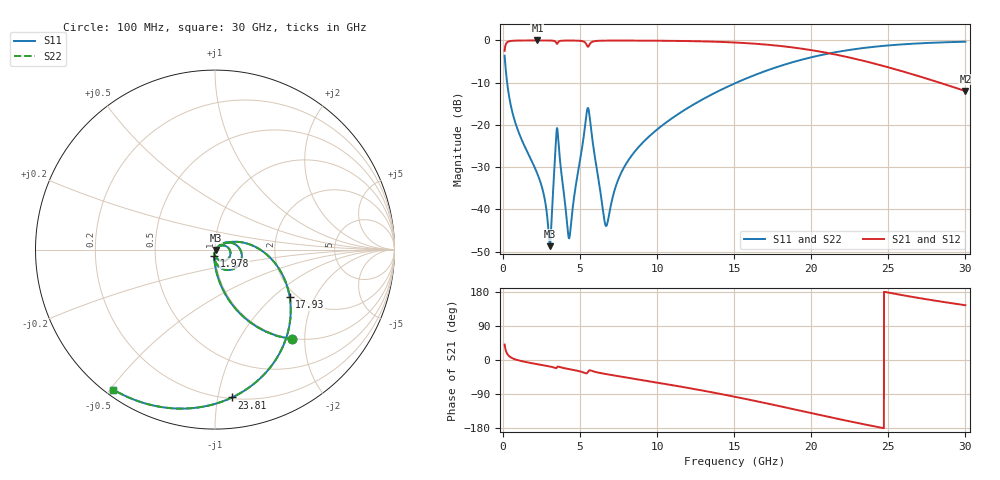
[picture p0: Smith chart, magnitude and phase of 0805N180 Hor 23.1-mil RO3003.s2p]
# GHz S MA R 50
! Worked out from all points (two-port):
!   3201 points, 100 MHz to 30 GHz, reference 50 ohm
!   highest |S21| = -0.02 dB at 2.23 GHz (marker M1); lowest = -12.0 dB at 30 GHz (marker M2)
!   |S21| within 3 dB of the highest: start of sweep to 21.11 GHz
!   lowest |S11| = -48.7 dB at 3.034 GHz (marker M3), VSWR 1.01, Z = 50.3 - j0.179 ohm
!   |S11| at or under -10 dB: 261.9 MHz to 15.15 GHz (14.89 GHz wide, 193 % of centre)
!   |S22| runs from -48.7 to -0.3 dB; largest |S21 - S12| = 0
!   S11 on the Smith chart (normalised r, x): 100 MHz: 0.98, -1.74; 1.978 GHz: 0.99, -0.07; 17.93 GHz: 1.84, -1.29; 23.81 GHz: 0.21, -1.10; 30 GHz: 0.02, -0.51
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0.1  0.6588 -49.3  0.752 40.6  0.752 40.6  0.6588 -49.3
0.3335938  0.2527 -77.1  0.967 12.7  0.967 12.7  0.2527 -77.1
0.7073438  0.1198 -86.7  0.9919 2.9  0.9919 2.9  0.1198 -86.7
1.978094  0.03354 -96.7  0.9978 -9.3  0.9978 -9.3  0.03354 -96.7
2.230375  0.02625 -97.4  0.9979 -11.1  0.9979 -11.1  0.02625 -97.4
3.033937  0.003665 -29.0  0.9963 -17.1  0.9963 -17.1  0.003665 -29.0
3.398344  0.05028 27.5  0.9661 -21.3  0.9661 -21.3  0.05028 27.5
3.501125  0.09161 -23.8  0.9085 -19.3  0.9085 -19.3  0.09161 -23.8
4.276656  0.004545 -26.6  0.9953 -24.0  0.9953 -24.0  0.004545 -26.6
5.089563  0.04838 40.8  0.9838 -31.1  0.9838 -31.1  0.04838 40.8
5.40725  0.1316 6.1  0.8972 -35.2  0.8972 -35.2  0.1316 6.1
5.55675  0.1494 -46.1  0.8564 -28.5  0.8564 -28.5  0.1494 -46.1
6.519156  0.008698 -71.0  0.9926 -36.0  0.9926 -36.0  0.008698 -71.0
6.706031  0.00637 -25.0  0.9935 -37.3  0.9935 -37.3  0.00637 -25.0
7.845969  0.03134 36.4  0.9946 -45.1  0.9946 -45.1  0.03134 36.4
10.06978  0.09037 27.0  0.9909 -60.0  0.9909 -60.0  0.09037 27.0
15.05  0.3105 -8.3  0.9435 -97.1  0.9435 -97.1  0.3105 -8.3
17.92788  0.4939 -32.5  0.861 -121.6  0.861 -121.6  0.4939 -32.5
20.03956  0.6331 -51.2  0.7646 -140.5  0.7646 -140.5  0.6331 -51.2
23.80509  0.8293 -83.4  0.5481 -172.8  0.5481 -172.8  0.8293 -83.4
25.01978  0.8719 -92.9  0.4786 177.7  0.4786 177.7  0.8719 -92.9
30  0.9644 -126.0  0.2512 144.5  0.2512 144.5  0.9644 -126.0
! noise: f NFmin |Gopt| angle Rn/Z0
0.1  0.000512  0.8815  0.9681  0.0009358
3.417  0.02897  0.9271  19.25  0.0857
6.743  0.01515  0.755  37.46  0.01123
10.06  0.01617  0.6818  54.4  0.007859
13.39  0.0207  0.6807  70.2  0.008548
16.7  0.02641  0.6962  84.82  0.009502
20.03  0.0338  0.722  98.53  0.01062
23.35  0.04377  0.7557  111.5  0.01194
26.67  0.05808  0.7958  124.2  0.01348
30  0.07989  0.8397  136.7  0.01504
